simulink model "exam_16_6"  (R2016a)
settings: Solver=VariableStepAuto  StartTime=0.0  StopTime=0.1  MaxStep=1e-4  RelTol=1e-3
libraries: powerlib x8

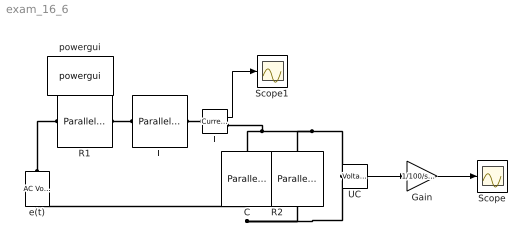
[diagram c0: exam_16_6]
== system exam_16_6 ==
  C : powerlib/Elements/Parallel RLC Branch  LConnTagsString=a  RConnTagsString=__new0  BranchType=C  Resistance=10  Inductance=1e-3  SetiL0=off  InitialCurrent=0  Capacitance=10e-6  Setx0=off  InitialVoltage=0  Measurements=None
  Gain : Gain  Gain=1/100/sqrt(2)
  IL : powerlib/Measurements/Current Measurement  PhasorSimulation=off  OutputType=Complex  PSBequivalent=0
  L : powerlib/Elements/Parallel RLC Branch  LConnTagsString=a  RConnTagsString=__new0  BranchType=L  Resistance=10  Inductance=0.5  SetiL0=off  InitialCurrent=0  Capacitance=1e-6  Setx0=off  InitialVoltage=0  Measurements=None
  R1 : powerlib/Elements/Parallel RLC Branch  LConnTagsString=a  RConnTagsString=__new0  BranchType=R  Resistance=10  Inductance=1e-3  SetiL0=off  InitialCurrent=0  Capacitance=1e-6  Setx0=off  InitialVoltage=0  Measurements=None
  R2 : powerlib/Elements/Parallel RLC Branch  LConnTagsString=a  RConnTagsString=__new0  BranchType=R  Resistance=1000  Inductance=1e-3  SetiL0=off  InitialCurrent=0  Capacitance=1e-6  Setx0=off  InitialVoltage=0  Measurements=None
  Scope : Scope
  Scope1 : Scope
  UC : powerlib/Measurements/Voltage Measurement  PhasorSimulation=off  OutputType=Complex  PSBequivalent=0
  e(t) : powerlib/Electrical Sources/AC Voltage Source  Amplitude=100*sqrt(2)  Phase=0  Frequency=50  SampleTime=0  Measurements=None  BusType=swing  Pref=10e3  Qref=0  Qmin=-inf  Qmax=+inf
  powergui : powerlib/powergui  Priority=1  SimulationMode=Continuous  SolverType=Tustin/Backward Euler (TBE)  SampleTime=50e-6  frequency=60  SPID=off  DisableSnubberDevices=off  DisableRonSwitches=off  DisableVfSwitches=off  SwTol=0  DisplayEquations=off  Interpol=off  ExternalGateDelay=off  methode=off  Ts=10  FunctionMessages=off  echomessages=off  HookPort=off  EnableUseOfTLC=off  x0status=blocks  frequencyindice=50  Pbase=100e6  ErrMax=1e-4  Iterations=50  UnitsV=kV  UnitsW=MW  buscounter=0  RestoreLinks=warning  ResistiveCurrentMeasurement=off  Frange=[0:2:500]  Ylog=off  Xlog=on  ShowGrid=off  save=off  variable=ZData  structure=0  ZoomFFT=off  StartTime=0.0  cycles=1  DisplayStyle=1  fundamental=60  FreqAxis=off  MaxFrequency=1000  frequencyindicesteady=1  RmsSteady=1  display=off
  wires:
  UC/1 -> Gain/1
  Gain/1 -> Scope/1
  IL/1 -> Scope1/1
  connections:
  L/LConn1 -- R1/RConn1
  e(t)/RConn1 -- R1/LConn1
  UC/LConn1 -- R2/LConn1 -- C/LConn1 -- IL/RConn1
  e(t)/LConn1 -- R2/RConn1 -- UC/LConn2 -- C/RConn1
  IL/LConn1 -- L/RConn1
